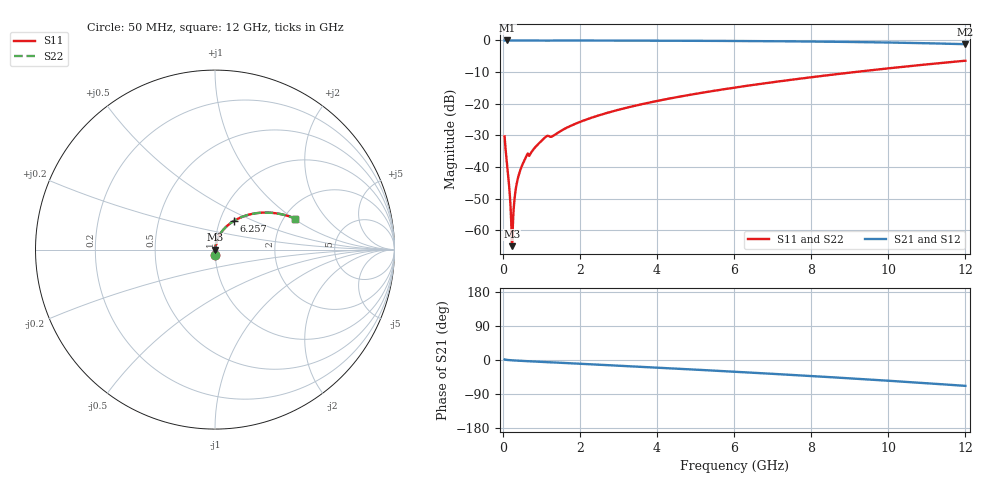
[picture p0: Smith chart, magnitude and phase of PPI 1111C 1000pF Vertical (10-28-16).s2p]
# GHz S MA R 50
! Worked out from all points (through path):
!   1601 points, 50 MHz to 12 GHz, reference 50 ohm
!   highest |S21| = 0.00 dB at 117.2 MHz (marker M1); lowest = -1.2 dB at 12 GHz (marker M2)
!   group delay of S21, straight-line fit = 15.7 ps
!   lowest |S11| = -65.0 dB at 244.2 MHz (marker M3), VSWR 1.00, Z = 50.1 + j0.00359 ohm
!   |S11| at or under -10 dB: start of sweep to 9.121 GHz
!   |S22| runs from -65.0 to -6.4 dB; largest |S21 - S12| = 0
!   S11 on the Smith chart (normalised r, x): 50 MHz: 1.00, -0.06; 6.257 GHz: 1.16, +0.38; 12 GHz: 2.29, +1.03
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0.05  0.03045 -87.8  0.9992 1.6  0.9992 1.6  0.03045 -87.8
0.08734375  0.01587 -88.0  0.9995 0.6  0.9995 0.6  0.01587 -88.0
0.1172187  0.01043 -87.5  0.9995 0.2  0.9995 0.2  0.01043 -87.5
0.1545625  0.006162 -85.8  0.9995 -0.2  0.9995 -0.2  0.006162 -85.8
0.199375  0.002678 -79.4  0.9995 -0.5  0.9995 -0.5  0.002678 -79.4
0.2217813  0.001333 -66.8  0.9994 -0.7  0.9994 -0.7  0.001333 -66.8
0.2441875  0.0005637 3.6  0.9994 -0.9  0.9994 -0.9  0.0005637 3.6
0.2815313  0.002008 71.6  0.9994 -1.1  0.9994 -1.1  0.002008 71.6
0.3338125  0.004272 80.0  0.9993 -1.4  0.9993 -1.4  0.004272 80.0
0.3935625  0.006622 82.3  0.9993 -1.8  0.9993 -1.8  0.006622 82.3
0.4831875  0.009882 83.3  0.9991 -2.3  0.9991 -2.3  0.009882 83.3
0.6101562  0.01465 82.4  0.9987 -3.0  0.9987 -3.0  0.01465 82.4
1.118031  0.03009 78.8  0.9966 -5.6  0.9966 -5.6  0.03009 78.8
1.297281  0.03082 77.6  0.9962 -6.3  0.9962 -6.3  0.03082 77.6
2.044156  0.0528 78.2  0.9969 -10.1  0.9969 -10.1  0.0528 78.2
2.910531  0.07762 74.2  0.9951 -14.6  0.9951 -14.6  0.07762 74.2
4.038312  0.1118 68.6  0.9915 -20.4  0.9915 -20.4  0.1118 68.6
6.025  0.1802 58.2  0.9807 -31.0  0.9807 -31.0  0.1802 58.2
6.256531  0.189 56.9  0.979 -32.3  0.979 -32.3  0.189 56.9
8.019156  0.2632 46.9  0.9611 -42.4  0.9611 -42.4  0.2632 46.9
10.01331  0.3631 34.6  0.9274 -54.8  0.9274 -54.8  0.3631 34.6
12  0.4785 21.2  0.8727 -68.2  0.8727 -68.2  0.4785 21.2
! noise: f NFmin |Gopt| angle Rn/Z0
0.05  0.0003805  0.8688  0.1919  0.0006238
1.372  0.005457  0.7634  4.713  0.004674
2.701  0.006687  0.6464  8.985  0.003563
4.031  0.008974  0.6162  13.16  0.004297
5.36  0.01122  0.5993  17.2  0.005047
6.682  0.01348  0.5907  21.08  0.005841
8.012  0.01584  0.5884  24.87  0.006733
9.341  0.01837  0.5915  28.56  0.007771
10.67  0.02113  0.5994  32.15  0.009016
12  0.02422  0.6118  35.69  0.01055
